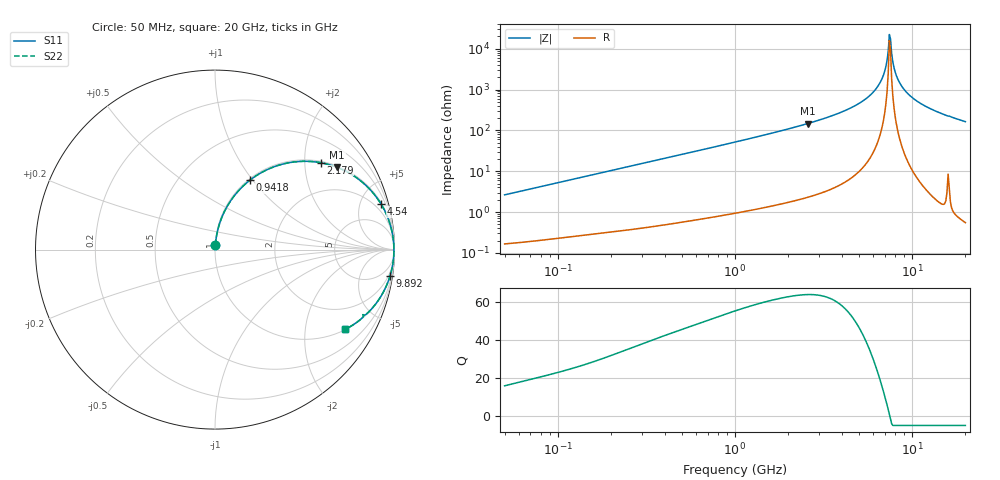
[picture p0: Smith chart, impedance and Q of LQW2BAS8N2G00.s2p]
!Murata Part Number: LQW2BAS8N2G00
!These Parameters are Measured in Series Mode Connection
!  o--[Z]--o
!Port1  Port2
!  o-------o
!Freq. Start=50[MHz] Stop=20[GHz], 401[Steps]
# Hz S RI R 50
!Freq.(Hz) S11(Real) S11(Imag) S21(Real) S21(Imag) S12(Real) S12(Imag) S22(Real) S22(Imag)
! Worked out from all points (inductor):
!   401 points, 50 MHz to 20 GHz, reference 50 ohm
!   read as one part in series: L = 8.36 nH near 51.52 MHz
!   highest Q = 63.9 at 2.569 GHz (marker M1), where L = 9.08 nH
!   self-resonance near 7.442 GHz
!   S11 on the Smith chart (normalised r, x): 50 MHz: 1.00, +0.05; 941.8 MHz: 1.02, +0.97; 2.179 GHz: 1.04, +2.40; 4.54 GHz: 1.14, +7.20; 9.892 GHz: 1, -13; 20 GHz: 1.01, -3.27
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5e7  0.00235 0.0262  0.9977 -0.0262  0.9977 -0.0262  0.00235 0.0262
1.364002e8  0.00762 0.0701  0.9924 -0.0701  0.9924 -0.0701  0.00762 0.0701
3.721004e8  0.0394 0.1828  0.9606 -0.1828  0.9606 -0.1828  0.0394 0.1828
9.418449e8  0.1953 0.3873  0.8047 -0.3873  0.8047 -0.3873  0.1953 0.3873
1e9  0.2148 0.4017  0.7852 -0.4017  0.7852 -0.4017  0.2148 0.4017
2.179053e9  0.5886 0.4843  0.4114 -0.4843  0.4114 -0.4843  0.5886 0.4843
2.569357e9  0.6797 0.4588  0.3203 -0.4588  0.3203 -0.4588  0.6797 0.4588
2.728004e9  0.7116 0.4453  0.2884 -0.4453  0.2884 -0.4453  0.7116 0.4453
4.539627e9  0.9243 0.2552  0.0757 -0.2552  0.0757 -0.2552  0.9243 0.2552
5.598765e9  0.9721 0.152  0.0279 -0.152  0.0279 -0.152  0.9721 0.152
6.406762e9  0.9895 0.0822  0.0105 -0.0822  0.0105 -0.0822  0.9895 0.0822
6.905011e9  0.9947 0.0428  0.00525 -0.0428  0.00525 -0.0428  0.9947 0.0428
7.114996e9  0.9959 0.0269  0.00405 -0.0269  0.00405 -0.0269  0.9959 0.0269
7.331367e9  0.9966 0.0111  0.00337 -0.0111  0.00337 -0.0111  0.9966 0.0111
7.442007e9  0.9968 0.00312  0.00322 -0.00312  0.00322 -0.00312  0.9968 0.00312
7.668323e9  0.9967 -0.0128  0.00329 0.0128  0.00329 0.0128  0.9967 -0.0128
8.020766e9  0.9956 -0.0366  0.00437 0.0366  0.00437 0.0366  0.9956 -0.0366
8.389408e9  0.9934 -0.0603  0.00659 0.0603  0.00659 0.0603  0.9934 -0.0603
9.041845e9  0.9871 -0.0998  0.0129 0.0998  0.0129 0.0998  0.9871 -0.0998
9.892087e9  0.9753 -0.1466  0.0247 0.1466  0.0247 0.1466  0.9753 -0.1466
1.314879e10  0.9069 -0.2869  0.0931 0.2869  0.0931 0.2869  0.9069 -0.2869
2e10  0.7269 -0.4439  0.2731 0.4439  0.2731 0.4439  0.7269 -0.4439
